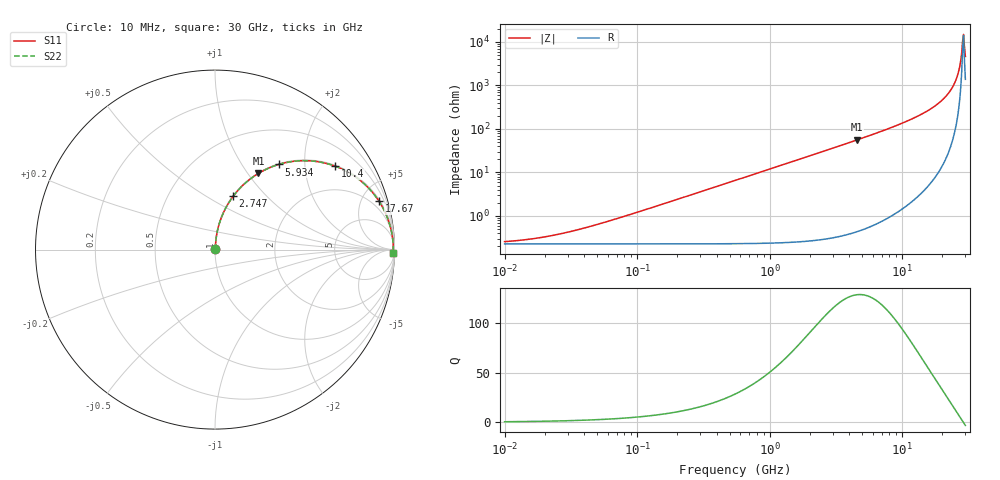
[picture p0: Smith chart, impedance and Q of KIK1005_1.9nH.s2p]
!version-3
!date-01.2023
!Series
# Hz S RI R 50
!Freq ReS11 ImS11 ReS21 ImS21 ReS12 ImS12 ReS22 ImS22
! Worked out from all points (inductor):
!   500 points, 10 MHz to 30 GHz, reference 50 ohm
!   read as one part in series: L = 1.9 nH near 57.48 MHz
!   highest Q = 128 at 4.59 GHz (marker M1), where L = 1.95 nH
!   self-resonance near 28.59 GHz
!   S11 on the Smith chart (normalised r, x): 10 MHz: 1.00, +0.00; 2.747 GHz: 1.01, +0.66; 5.934 GHz: 1.01, +1.48; 10.4 GHz: 1.03, +2.85; 17.67 GHz: 1.15, +6.72; 30 GHz: 29, -88
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1e7  0.00228 0.00119  0.9977 -0.00119  0.9977 -0.00119  0.00228 0.00119
1.96184e7  0.00228 0.00233  0.9977 -0.00233  0.9977 -0.00233  0.00228 0.00233
3.848815e7  0.0023 0.00457  0.9977 -0.00457  0.9977 -0.00457  0.0023 0.00457
1.457759e8  0.00258 0.0173  0.9974 -0.0173  0.9974 -0.0173  0.00258 0.0173
5.521343e8  0.0066 0.0653  0.9934 -0.0653  0.9934 -0.0653  0.0066 0.0653
2.091238e9  0.0615 0.2349  0.9385 -0.2349  0.9385 -0.2349  0.0615 0.2349
2.747025e9  0.1009 0.2966  0.8991 -0.2966  0.8991 -0.2966  0.1009 0.2966
4.590334e9  0.2418 0.4243  0.7582 -0.4243  0.7582 -0.4243  0.2418 0.4243
5.933831e9  0.3546 0.4744  0.6454 -0.4744  0.6454 -0.4744  0.3546 0.4744
7.920679e9  0.5108 0.4954  0.4892 -0.4954  0.4892 -0.4954  0.5108 0.4954
1.040451e10  0.6687 0.4652  0.3313 -0.4652  0.3313 -0.4652  0.6687 0.4652
1.388829e10  0.8189 0.3776  0.1811 -0.3776  0.1811 -0.3776  0.8189 0.3776
1.766735e10  0.9135 0.27  0.0865 -0.27  0.0865 -0.27  0.9135 0.27
2.107761e10  0.9604 0.1782  0.0396 -0.1782  0.0396 -0.1782  0.9604 0.1782
2.396441e10  0.9818 0.1073  0.0182 -0.1073  0.0182 -0.1073  0.9818 0.1073
2.514614e10  0.987 0.0802  0.013 -0.0802  0.013 -0.0802  0.987 0.0802
2.638614e10  0.9907 0.0529  0.00927 -0.0529  0.00927 -0.0529  0.9907 0.0529
2.724659e10  0.9924 0.0346  0.00763 -0.0346  0.00763 -0.0346  0.9924 0.0346
2.81351e10  0.9933 0.0163  0.00668 -0.0163  0.00668 -0.0163  0.9933 0.0163
2.859017e10  0.9935 0.00717  0.00646 -0.00717  0.00646 -0.00717  0.9935 0.00717
2.95225e10  0.9935 -0.0112  0.00652 0.0112  0.00652 0.0112  0.9935 -0.0112
3e10  0.9932 -0.0203  0.0068 0.0203  0.0068 0.0203  0.9932 -0.0203
